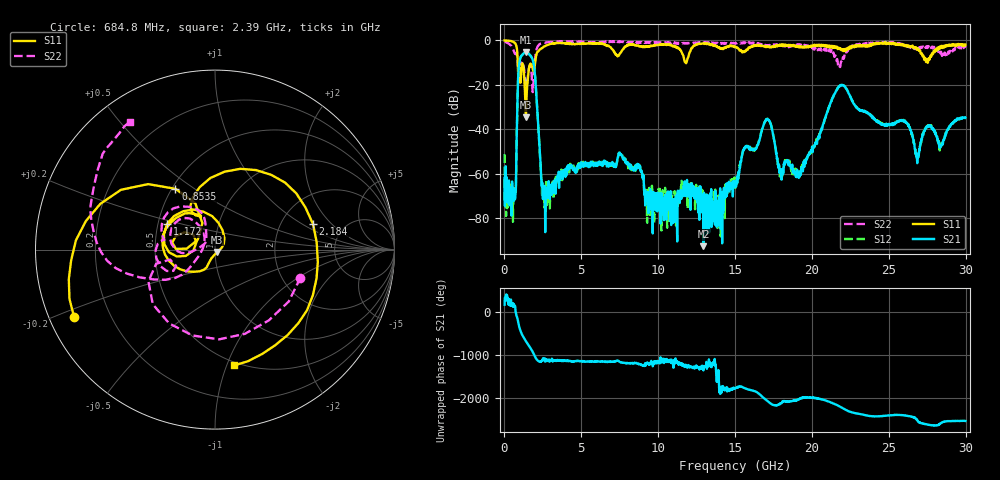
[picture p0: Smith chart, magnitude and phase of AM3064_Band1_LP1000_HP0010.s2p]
# Hz S DB R 50.0
!freq dBS11 angS11 dBS21 angS21 dBS12 angS12 dBS22 angS22
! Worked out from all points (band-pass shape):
!   1600 points, 10 MHz to 29.98 GHz, reference 50 ohm
!   highest |S21| = -5.23 dB at 1.397 GHz (marker M1); lowest = -92.6 dB at 12.94 GHz (marker M2)
!   |S21| within 3 dB of the highest: 1.023 GHz to 1.811 GHz (788 MHz wide, 55.6 % of centre)
!   lowest |S11| = -34.6 dB at 1.397 GHz (marker M3), VSWR 1.04, Z = 51.2 - j1.41 ohm
!   |S11| at or under -10 dB: 866 MHz to 1.997 GHz (1.131 GHz wide, 79 % of centre); 11.7881 GHz to 11.83865 GHz (50.55 MHz wide, 0.428 % of centre); 27.52396 GHz to 27.53758 GHz (13.63 MHz wide, 0.0495 % of centre)
!   |S22| runs from -23.6 to -0.4 dB; largest |S21 - S12| = 0.0069
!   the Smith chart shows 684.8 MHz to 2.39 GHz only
!   S11 on the Smith chart (normalised r, x): 684.8 MHz: 0.07, -0.22; 853.5 MHz: 0.52, +0.42; 1.172 GHz: 0.56, +0.18; 2.184 GHz: 3.02, +1.26; 2.39 GHz: 0.47, -1.07
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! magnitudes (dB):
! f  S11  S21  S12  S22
! 10 MHz  0.0  -61.9  -51.2  -0.4
! 234.9 MHz  -0.1  -66.6  -70.9  -1.3
! 684.8 MHz  -1.2  -71.5  -67.5  -6.0
! 853.5 MHz  -7.9  -25.0  -24.9  -9.4
! 1.172 GHz  -10.4  -6.5  -6.4  -9.5
! 1.397 GHz  -34.6  -5.2  -5.2  -22.6
! 1.866 GHz  -13.6  -9.4  -9.4  -21.1
! 2.184 GHz  -5.0  -36.6  -36.8  -2.5
! 2.39 GHz  -3.7  -62.3  -61.6  -1.4
! 2.69 GHz  -2.3  -69.2  -67.3  -0.9
! 5.015 GHz  -1.3  -55.9  -55.8  -0.6
! 7.545 GHz  -5.6  -51.3  -51.7  -0.7
! 10 GHz  -2.0  -74.3  -71.1  -0.9
! 12.94 GHz  -1.5  -92.6  -72.4  -1.0
! 15 GHz  -2.9  -64.1  -65.1  -1.4
! 17.07 GHz  -2.7  -35.4  -35.3  -2.2
! 18 GHz  -2.0  -59.0  -59.6  -2.4
! 19.99 GHz  -2.8  -49.5  -49.3  -3.0
! 21.88 GHz  -4.0  -20.3  -20.2  -9.8
! 25 GHz  -1.0  -37.6  -38.1  -1.1
! 26.85 GHz  -4.3  -55.3  -52.3  -3.1
! 29.98 GHz  -1.9  -34.8  -34.7  -3.2
